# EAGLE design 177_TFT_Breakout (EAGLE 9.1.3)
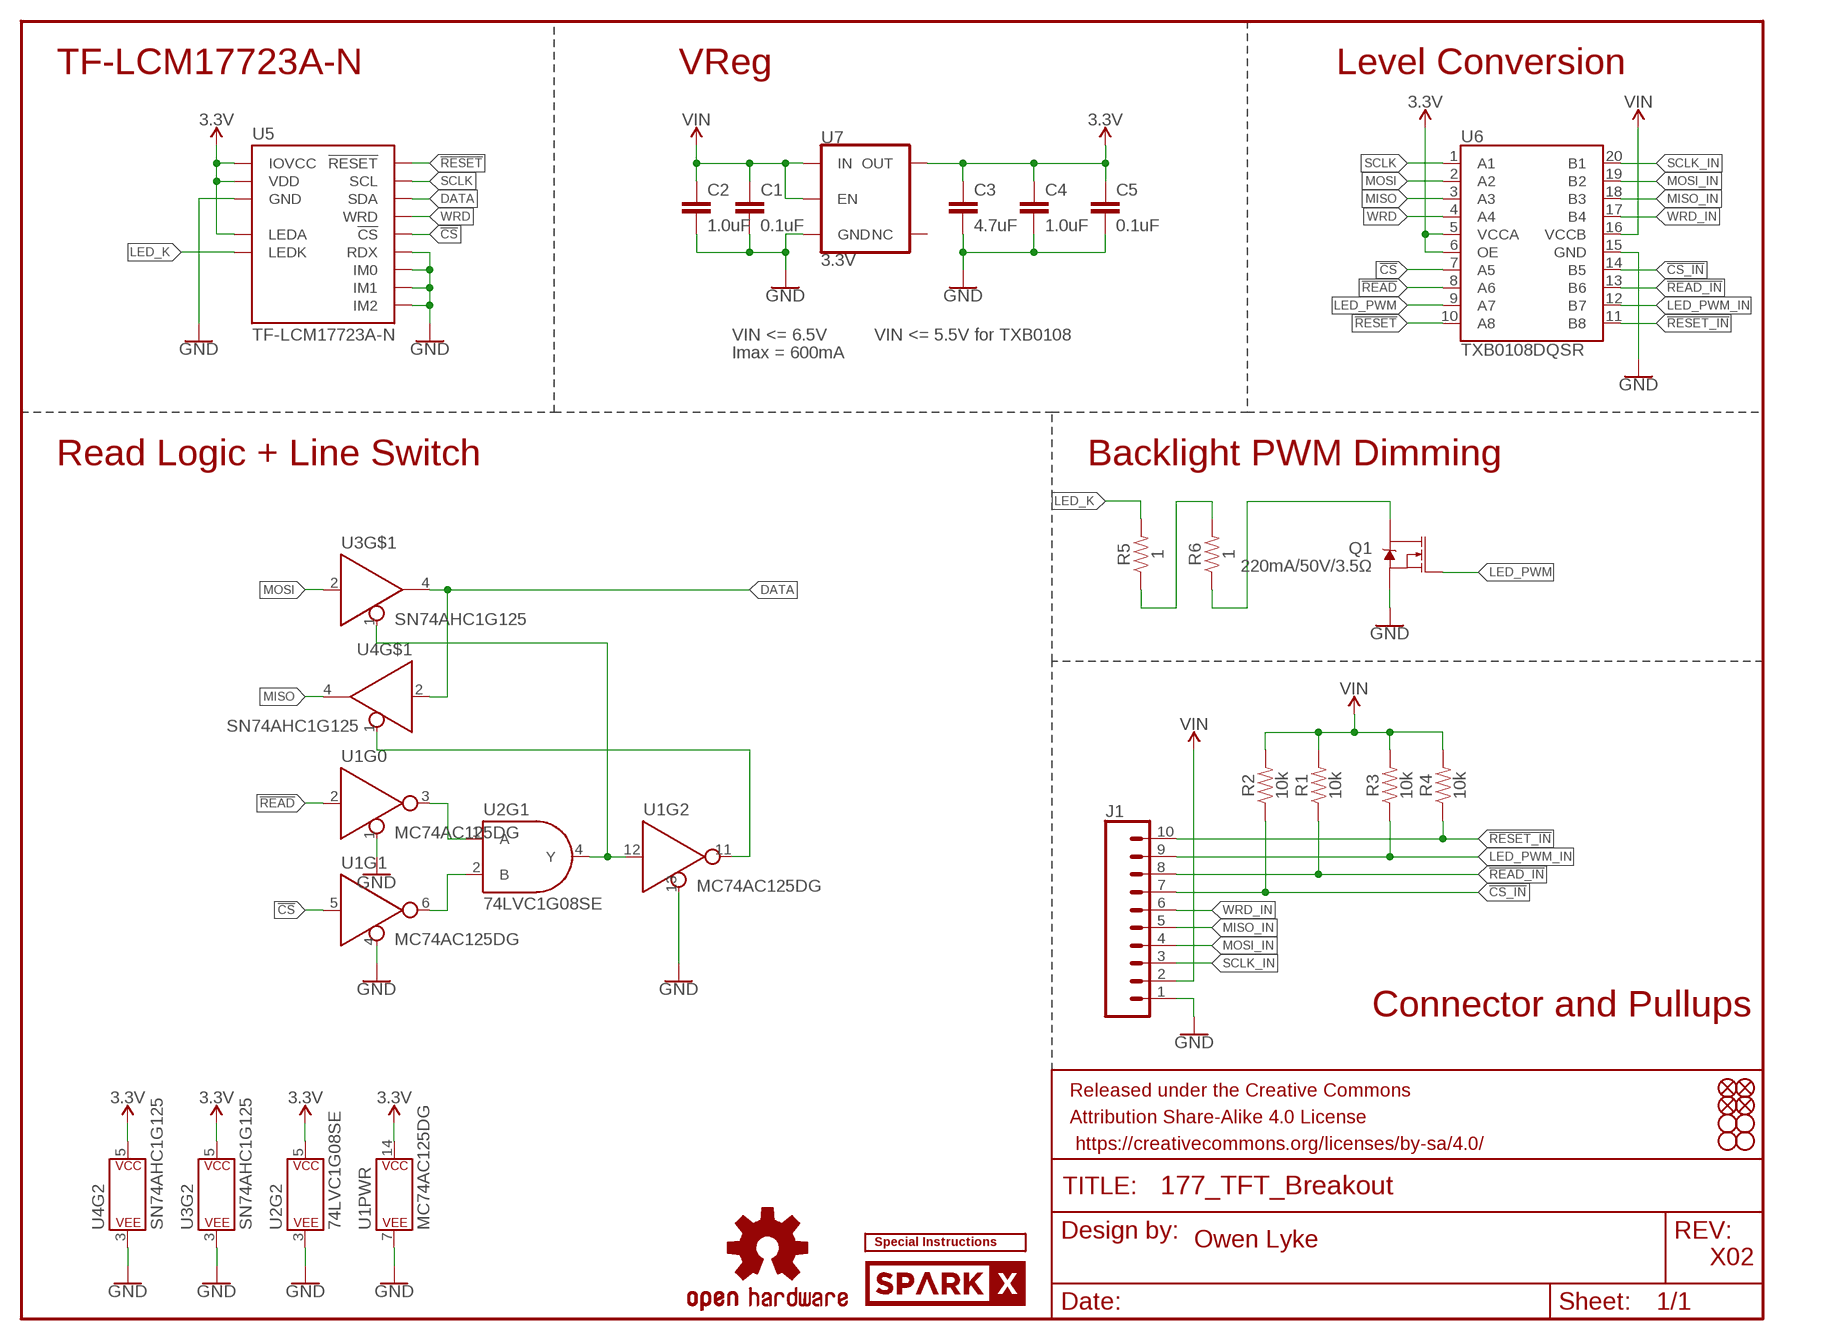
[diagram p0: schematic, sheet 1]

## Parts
C1  0.1uF  0.1UF-0603-100V-10%  [0603]
C2  1.0uF  1.0UF-0603-16V-10%  [0603]
C3  4.7uF  4.7UF-0603-6.3V-(10%)  [0603]
C4  1.0uF  1.0UF-0603-16V-10%  [0603]
C5  0.1uF  0.1UF-0603-100V-10%  [0603]
FD1  FIDUCIAL1X2  [FIDUCIAL-1X2]
FD2  FIDUCIAL1X2  [FIDUCIAL-1X2]
FD3  FIDUCIAL1X2  [FIDUCIAL-1X2]
FD4  FIDUCIAL1X2  [FIDUCIAL-1X2]
FRAME1  FRAME-LETTER  [CREATIVE_COMMONS]
H1  STAND-OFF  [STAND-OFF]
H2  STAND-OFF  [STAND-OFF]
H3  STAND-OFF  [STAND-OFF]
H4  STAND-OFF  [STAND-OFF]
J1  CONN_10NO_SILK_PTH_FEMALE  [1X10_NO_SILK]
LOGO1  OSHW-LOGOMINI  [OSHW-LOGO-MINI]
Q1  220mA/50V/3.5Ω  MOSFET-NCH-BSS138  [SOT23-3]
R1  10k  10KOHM-0603-1/10W-1%  [0603]
R2  10k  10KOHM-0603-1/10W-1%  [0603]
R3  10k  10KOHM-0603-1/10W-1%  [0603]
R4  10k  10KOHM-0603-1/10W-1%  [0603]
R5  1  1OHM-0603-1/10W-1%  [0603]
R6  1  1OHM-0603-1/10W-1%  [0603]
U1  MC74AC125DG  74AC125DG  [SO14]
U2  74LVC1G08SE  74LVC08SE  [SOT23-5]
U3  SN74AHC1G125  74AHC1G125D  [SOT23-5]
U4  SN74AHC1G125  74AHC1G125D  [SOT23-5]
U5  TF-LCM17723A-N  TF-LCM17723A-N-BOTTOM_CONTACTS  [FPC05040-17204]
U6  TXB0108DQSR  TXB0108  [UFDFN-20]
U7  3.3V  V_REG_AP2112K-3.3V  [SOT23-5]
U$26  SPECIAL_INSTRUCTIONS-ORDERING  [ORDERING_INSTRUCTIONS]
U$34  SPARKX-LOGO2  [SPARKX-TINY]

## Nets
3.3V: C3.1 C4.1 C5.1 U1.14(PWR:P$V+) U2.5(P$V+) U3.5(P$V+) U4.5(P$V+) U5.P$8(LEDA) U5.P$9(VDD) U5.P$10(IOVCC) U6.5(VCCA) U6.6(OE) U7.5(OUT)
!CS: U1.5(A) U5.P$35(!CS) U6.7(A5)
!CS_IN: J1.7 R2.1 U6.14(B5)
!READ: U1.2(A) U6.8(A6)
!READ_IN: J1.8 R1.1 U6.13(B6)
!RESET: U5.P$37(!RESET) U6.10(A8)
!RESET_IN: J1.10 R4.1 U6.11(B8)
DATA: U3.4(Y) U4.2(A) U5.P$29(SDA) U5.P$31(SDA)
GND: C1.2 C2.2 C3.2 C4.2 C5.2 J1.1 Q1.2(S) U1.1(!EN) U1.4(!EN) U1.7(PWR:P$V-) U1.13(!EN) U2.3(P$V-) U3.3(P$V-) U4.3(P$V-) U5.P$1(GND) U5.P$2(GND) U5.P$3(GND) U5.P$4(GND) U5.P$11(GND) U5.P$12(GND) U5.P$13(GND) U5.P$32(RDX) U5.P$38(IM0) U5.P$39(IM1) U5.P$40(IM2) U6.15(GND) U7.2(GND)
LED_K: R5.2 U5.P$6(LEDK) U5.P$7(LEDK)
LED_PWM: Q1.1(G) U6.9(A7)
LED_PWM_IN: J1.9 R3.1 U6.12(B7)
MISO: U4.4(Y) U6.3(A3)
MISO_IN: J1.5 U6.18(B3)
MOSI: U3.2(A) U6.2(A2)
MOSI_IN: J1.4 U6.19(B2)
N$1: U1.6(Y) U2.2(B)
N$2: U1.3(Y) U2.1(A)
N$3: U1.12(A) U2.4(Y) U3.1(!EN)
N$4: R5.1 R6.2
N$5: Q1.3(D) R6.1
N$8: U1.11(Y) U4.1(!EN)
SCLK: U5.P$34(SCL) U6.1(A1)
SCLK_IN: J1.3 U6.20(B1)
VIN: C1.1 C2.1 J1.2 R1.2 R2.2 R3.2 R4.2 U6.16(VCCB) U7.1(IN) U7.3(EN)
WRD: U5.P$33(WRD) U6.4(A4)
WRD_IN: J1.6 U6.17(B4)
Unconnected: U1.8(Y) U1.9(A) U1.10(!EN) U7.4(NC)

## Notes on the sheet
- TF-LCM17723A-N | VReg | Level Conversion
- VIN <= 6.5V | VIN <= 5.5V for TXB0108
- Imax = 600mA
- Read Logic + Line Switch | Backlight PWM Dimming
- Connector and Pullups
- Owen Lyke
- X02

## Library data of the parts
C1 C5 = SparkFun-Capacitors:0.1UF: 0.1µF ceramic capacitors; PROD_ID: CAP-08390
C2 C4 = SparkFun-Capacitors:1.0UF: 1µF ceramic capacitors; PROD_ID: CAP-00868
C3 = SparkFun-Capacitors:4.7UF: 4.7µF ceramic capacitors; PROD_ID: CAP-08280
FD1-FD4 = SparkFun-Aesthetics:FIDUCIAL: Fiducial Alignment Points
FRAME1 = SparkFun-Aesthetics:FRAME-LETTER: Schematic Frame - Letter
H1-H4 = SparkFun-Hardware:STAND-OFF: Stand Off
J1 = SparkFun-Connectors:CONN_10: Multi connection point. Often used as Generic Header-pin footprint for 0.1 inch spaced/style header connections On any of the 0.1 inch spaced packages, you can populate with these: Break Away Headers - Straight (PRT-00116) Break Away Male Headers - Right Angle (PRT-00553) Female Headers (PRT-00115)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; PROD_ID: CONN-11563
LOGO1 = SparkFun-Aesthetics:OSHW-LOGO: Open-Source Hardware (OSHW) Logo
Q1 = SparkFun-DiscreteSemi:MOSFET-NCH: N-channel MOSFETs Voltage controlled devices that allow control of high current outputs. SparkFun Products: SparkFun OpenScale SparkFun Digital Sandbox SparkFun Monster Moto Shield SparkFun MOSFET Power Controller; PROD_ID: TRANS-00830
R1-R4 = SparkFun-Resistors:10KOHM: 10kΩ resistor; PROD_ID: RES-00824
R5 R6 = SparkFun-Resistors:1OHM: 1Ω resistor; PROD_ID: RES-08269
U1 = SparkFun-IC-Logic:74*125: Quad inverter with enable BUFF TRI-ST QD N-INV 14SOIC SparkFun Products Pocket AVR Programmer (PGM-09825) SparkFun Line Follower Array (SEN-13582); PROD_ID: IC-08880
U2 = SparkFun-IC-Logic:74*08: Single AND gate IC GATE AND SNGL 2INPUT SOT353 SparkFun Products SparkFun LogicBlocks Kit (KIT-11006) SparkFun RedBot Mainboard (ROB-12097); PROD_ID: IC-10841
U3 U4 = SparkFun-IC-Logic:74*1G125: Single buffer Buffers & Line Drivers Tri-State Single Bus SOT-23-5 Datasheet SparkFun Products SparkFun SAMD21 Mini Breakout (DEV-13664) SparkFun SAMD21 Dev Breakout (DEV-13672) SparkFun MIDI Shield (DEV-12898) SparkFun WiFi Shield - CC3000 (DEV-12071); PROD_ID: IC-11920
U5 = all_displays:TF-LCM17723A-N
U6 = SparkFun-IC-Comms:TXB0108: 8-Bit Bi-Directional Level Shifter 1.2V-3.6V (VCCA) to 1.65V-5.5V (VCCB) bi-directional level shifter with auto direction sensing. Max data rate - VCCA 1.2V: 20Mbps (50ns), VCCA 3.3V: 100Mbps (10ns) Digikey: 296-27217-1-ND (20-UFDFN) SparkFun Products SparkFun GPS Logger Shield (GPS-13750) SparkFun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; PROD_ID: IC-12292
U7 = SparkFun-IC-Power:V_REG_AP2112: AP2112 - 600mA CMOS LDO Regulator w/ Enable The AP2112 is CMOS process low dropout linear regulator with enable function, the regulator delivers a guaranteed 600mA (min.) continuous load current. Features Output Voltage Accuracy: ±1.5% Output Current: 600mA (Min.) Foldback Short Current Protection: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; PROD_ID: VREG-12457
U$26 = SparkFun-Aesthetics:SPECIAL_INSTRUCTIONS: Special Ordering/Production Instructions Alert
U$34 = SparkX:SPARKX-LOGO

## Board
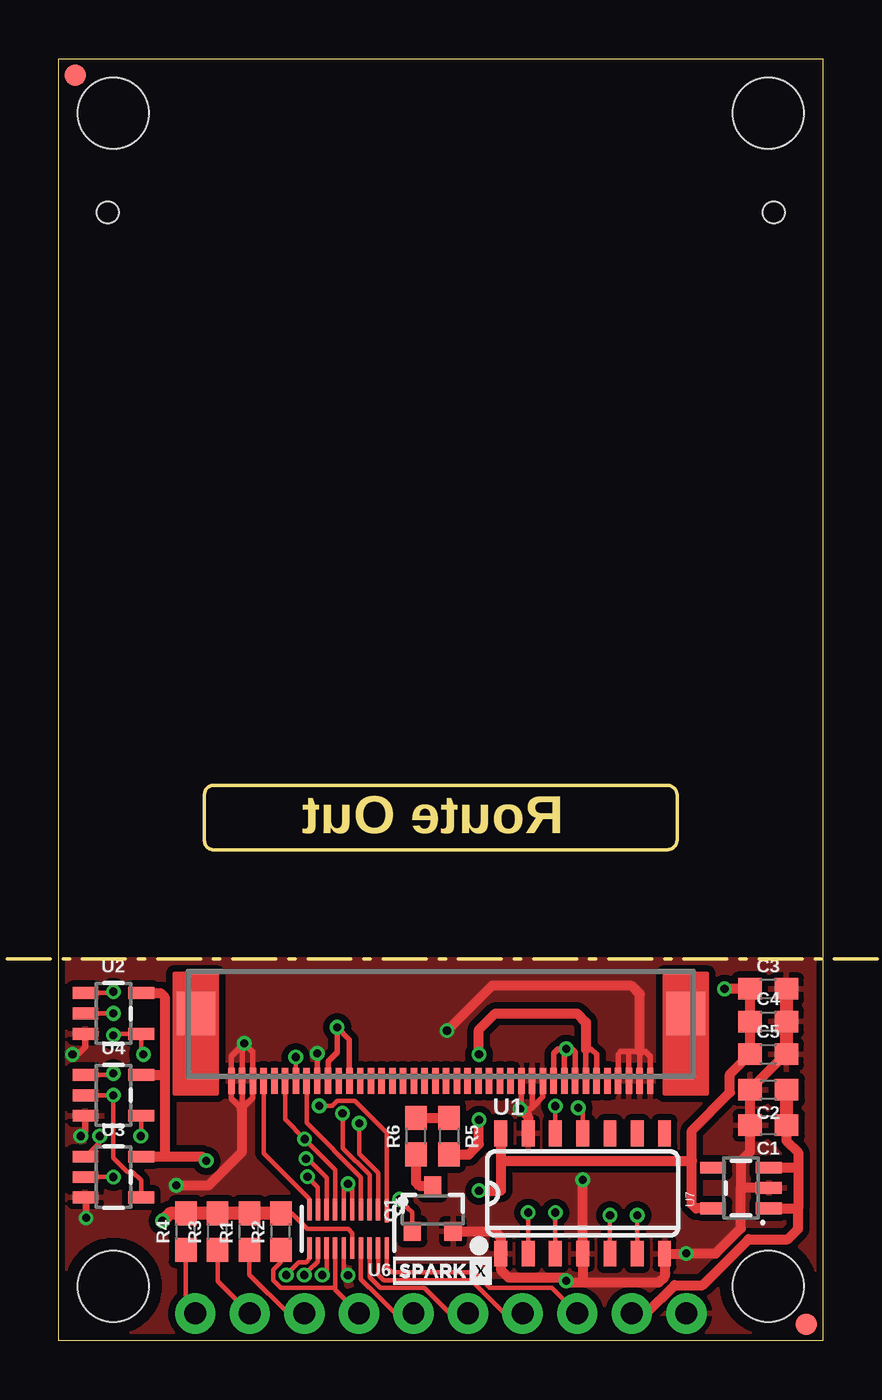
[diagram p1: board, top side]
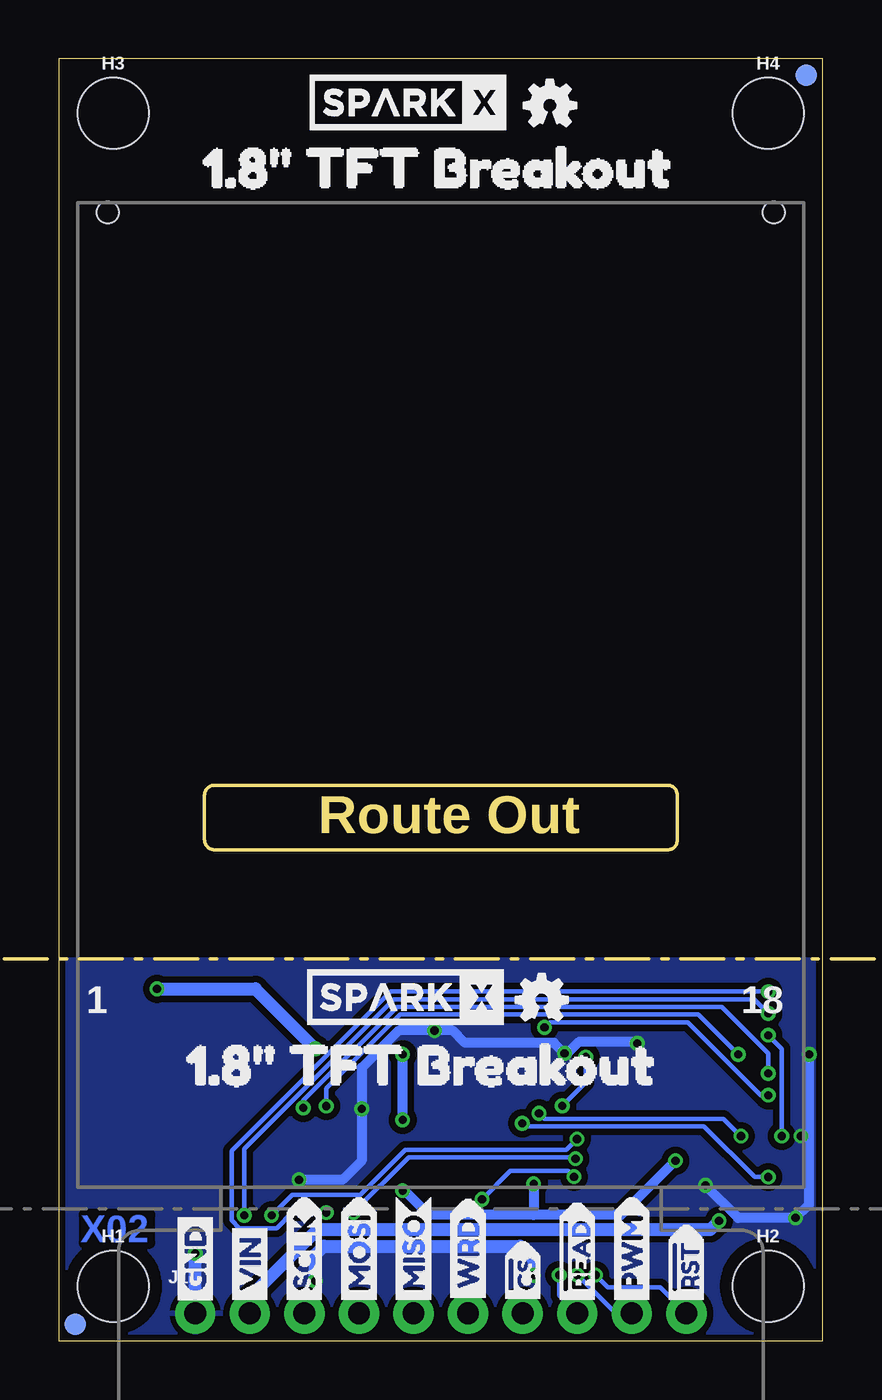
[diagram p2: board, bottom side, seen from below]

Size 35.56 x 59.69 mm. Coordinates in mm from the lower left corner, seen from the top.
Outline: 35.56,0 0,0 0,59.69 35.56,59.69 35.56,0
Copper layers (1*16): Top 0.035mm / dielectric 1.5mm / Bottom 0.035mm
Design rules "SparkFun-2-layer-PCBWay-LIMIT": minimum track width 6mil, minimum drill 0.3mm, track to track 6mil, track to pad 6mil, pad to pad 6mil, via to via 6mil, smd to smd 6mil, copper to edge 6mil, drill to drill 6mil, minimum pad ring 6mil, minimum via ring 6mil, stop-mask expansion 4mil, vias tented up to drill 25mil, thermal gap 10mil
Milling: 31 lines

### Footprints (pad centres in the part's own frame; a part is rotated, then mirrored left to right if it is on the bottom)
0603 = smd 1.1 x 1: 1 -0.85,0; 2 0.85,0
FIDUCIAL-1X2 = smd 1 x 1: 1 0,0
STAND-OFF = hole 3.302: 0,0
1X10_NO_SILK = drill 1.016 pad 1.88: 1 0,0; 2 2.54,0; 3 5.08,0; 4 7.62,0; 5 10.16,0; 6 12.7,0; 7 15.24,0; 8 17.78,0; 9 20.32,0; 10 22.86,0
SOT23-3 = smd 0.8 x 0.9: 1 -0.95,-1; 2 0.95,-1; 3 0,1.1
SO14 = smd 0.6 x 1.2: 1 -3.175,-2.8; 2 -1.905,-2.8; 3 -0.635,-2.8; 4 0.635,-2.8; 5 1.905,-2.8; 6 3.175,-2.8; 7 4.445,-2.8; 8 4.445,2.8; 9 3.175,2.8; 10 1.905,2.8; 11 0.635,2.8; 12 -0.635,2.8; 13 -1.905,2.8; 14 -3.175,2.8
SOT23-5 = smd 0.55 x 1.2: 1 -0.95,-1.3; 2 0,-1.3; 3 0.95,-1.3; 4 0.95,1.3; 5 -0.95,1.3
FPC05040-17204 = smd 0.3 x 1.2: P$1 -9.75,0.6; P$2 -9.25,0.6; P$3 -8.75,0.6; P$4 -8.25,0.6; P$5 -7.75,0.6; P$6 -7.25,0.6; P$7 -6.75,0.6; P$8 -6.25,0.6; P$9 -5.75,0.6; P$10 -5.25,0.6; P$11 -4.75,0.6; P$12 -4.25,0.6; P$13 -3.75,0.6; P$14 -3.25,0.6; P$15 -2.75,0.6; P$16 -2.25,0.6; P$17 -1.75,0.6; P$18 -1.25,0.6; P$19 -0.75,0.6; P$20 -0.25,0.6; P$21 0.25,0.6; P$22 0.75,0.6; P$23 1.25,0.6; P$24 1.75,0.6; P$25 2.25,0.6; P$26 2.75,0.6; P$27 3.25,0.6; P$28 3.75,0.6; P$29 4.25,0.6; P$30 4.75,0.6; P$31 5.25,0.6; P$32 5.75,0.6; P$33 6.25,0.6; P$34 6.75,0.6; P$35 7.25,0.6; P$36 7.75,0.6; P$37 8.25,0.6; P$38 8.75,0.6; P$39 9.25,0.6; P$40 9.75,0.6 | smd 1.8 x 2: P$41 -11.4,-2.55; P$42 11.4,-2.55
UFDFN-20 = smd 0.2 x 1.1: 1 -1.8,-0.85 | smd 0.2 x 1: 2 -1.4,-0.9; 3 -1,-0.9; 4 -0.6,-0.9; 5 -0.2,-0.9; 6 0.2,-0.9; 7 0.6,-0.9; 8 1,-0.9; 9 1.4,-0.9; 10 1.8,-0.9; 11 1.8,0.9; 12 1.4,0.9; 13 1,0.9; 14 0.6,0.9; 15 0.2,0.9; 16 -0.2,0.9; 17 -0.6,0.9; 18 -1,0.9; 19 -1.4,0.9; 20 -1.8,0.9
TF-LCM17723A-N_FLAT = hole 1: -15.5,75.4; 15.5,75.4

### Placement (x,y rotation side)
C1  33.02,10.03 180 top
C2  33.02,11.68 180 top
C3  33.02,16.38 0 top
C4  33.02,14.86 0 top
C5  33.02,13.34 0 top
FD1  34.8,0.76 0 bottom
FD2  0.76,58.93 0 bottom
FD3  34.8,0.76 0 top
FD4  0.76,58.93 0 top
FRAME1  not placed on the board
H1  33.02,2.54 0 bottom
H2  2.54,2.54 0 bottom
H3  33.02,57.15 0 bottom
H4  2.54,57.15 0 bottom
J1  29.21,1.27 0 bottom
LOGO1  12.7,57.53 0 bottom
LOGO2  OSHW-LOGOMINI  [OSHW-LOGO-MINI]  13.08,15.88 0 bottom
Q1  17.4,6.1 0 top
R1  8.86,5.08 90 top
R2  10.34,5.08 90 top
R3  7.39,5.08 90 top
R4  5.92,5.08 90 top
R5  18.16,9.53 270 top
R6  16.64,9.53 90 top
U1  23.75,6.86 0 top
U2  2.54,15.24 270 top
U3  2.54,7.62 270 top
U4  2.54,11.43 270 top
U5  17.78,12.7 180 top
U6  13.46,5.21 180 top
U7  31.75,7.11 90 top
U$1  [TF-LCM17723A-N_FLAT]  17.78,-22.86 0 bottom
U$3  [VIN2]  26.67,1.4 90 bottom
U$4  [GND1]  29.21,1.4 90 bottom
U$5  [MOSI8]  21.59,1.4 90 bottom
U$6  [MISO9]  19.05,1.4 90 bottom
U$7  [PWM8]  8.89,1.4 90 bottom
U$8  [#READ7]  11.43,1.27 90 bottom
U$9  [#CS6]  13.97,1.27 90 bottom
U$10  [WRD9]  16.51,1.52 90 bottom
U$11  [SCLK7]  24.13,1.4 90 bottom
U$12  [#RST2]  6.35,1.27 90 bottom
U$13  [SPARKX-MEDIUM]  19.3,57.66 0 bottom
U$14  [1#8#_TFT_BREAKOUT10]  30.48,54.61 0 bottom
U$15  [1#8#_TFT_BREAKOUT10]  31.24,12.83 0 bottom
U$26  not placed on the board
U$34  17.86,3.25 0 top
U$51  [SPARKX-MEDIUM]  19.43,16 0 bottom

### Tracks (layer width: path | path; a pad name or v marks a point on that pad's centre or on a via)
3.3V  (via drill 0.38)
  Top 0.203: U6.5 13.66,7.1 v13.46,7.3 13.26,7.11 U6.6
  Top 0.254: U5.P$10 23.03,13.38 23.24,13.59 v23.62,13.59 | U5.P$9 23.53,13.5 v23.62,13.59 | v23.62,13.59 23.88,13.59 24.03,13.44 U5.P$8
  Top 0.457: v30.99,16.38 C3.1 C4.1 C5.1 31.24,12.4 31.24,11.56 29.46,9.78 29.46,8.38 | v6.86,8.38 6.67,8.57 4.95,8.57 | 4.95,8.57 U3.5 | U2.5 4.74,16.19 4.92,16 4.92,12.32 | 4.92,12.32 4.92,8.6 4.95,8.57 | U4.5 4.86,12.38 4.92,12.32 | 29.46,8.38 29.46,6.35 29.65,6.16 U7.5 | U1.14 20.57,8.38 | 20.57,8.38 20.57,6.99 v19.56,6.99 | 20.57,8.38 29.46,8.38
  Bottom 0.457: v19.56,6.99 19.52,7.03 18.34,5.86 13.46,5.86 | v6.86,8.38 9.38,5.86 13.46,5.86 | v13.46,7.3 13.46,5.86
  Bottom 0.61: v30.99,16.38 26.42,16.38 v23.62,13.59
!CS  (via drill 0.38)
  Top 0.203: v25.65,5.84 U1.5 | U5.P$35 10.53,10.3 v11.44,9.39 12.86,7.97 U6.7
  Bottom 0.203: v25.65,5.84 24.7,6.79 21.52,6.79 19.43,8.89 11.94,8.89 v11.44,9.39
!CS_IN
  Top 0.203: U6.14 12.86,2.54 | 12.86,2.54 12.86,2.38 J1.7 | 12.86,2.54 12.79,2.46 10.34,2.46 9.99,2.81 9.99,3.31 10.34,3.66 R2.1
!READ  (via drill 0.38)
  Top 0.203: v21.84,5.97 U1.2 | U6.8 12.46,7.6 11.58,8.47 v11.51,8.47
  Bottom 0.203: v21.84,5.97 19.28,8.53 11.57,8.53 v11.51,8.47
!READ_IN  (via drill 0.38)
  Top 0.203: R1.1 8.87,3.07 10.67,1.27 J1.8 | U6.13 12.46,3.26 v12.27,3.06
  Bottom 0.203: v12.27,3.06 12.27,2.1 J1.8
!RESET
  Top 0.203: U6.10 11.66,6.6 9.53,8.74 U5.P$37
!RESET_IN  (via drill 0.38)
  Top 0.203: J1.10 5.92,1.7 R4.1 | U6.11 11.66,3.81 11.52,3.66 11.18,3.66 v10.58,3.06
  Bottom 0.203: J1.10 7.56,2.48 10,2.48 v10.58,3.06
DATA  (via drill 0.38)
  Top 0.203: U4.2 v2.54,11.43 2.54,8.51 3.17,7.87 3.43,7.87 3.84,7.46 U3.4
  Top 0.254: U5.P$29 13.53,14.02 v12.95,14.59 12.95,13.43 12.53,13 U5.P$31
  Bottom 0.203: v2.54,11.43 2.88,11.43 6.28,14.83 12.71,14.83 v12.95,14.59
GND  (via drill 0.38)
  Top 0.203: U6.15 13.26,3.25 v13.46,3.05 | v12.03,13.37 v12.02,13.38
  Top 0.254: 26.54,13.46 26.16,13.46 26.03,13.33 U5.P$4 | 26.54,13.46 27.05,13.46 | 27.05,13.46 27.3,13.46 27.53,13.24 U5.P$1 | 27.05,13.46 27.03,13.44 U5.P$2 | U5.P$13 21.53,10.86 v21.46,10.79 21.97,10.79 22.03,10.85 | U5.P$11 22.53,11.35 22.03,10.85 | U5.P$12 22.03,10.85 | U5.P$32 v12.03,13.37 | v8.64,13.84 8.03,13.24 U5.P$40 8.03,11.27 8.51,10.79 8.53,10.82 | v8.64,13.84 9.03,13.45 U5.P$38 9.03,11.32 8.53,10.82 | v8.64,13.84 8.53,13.74 U5.P$39 8.53,10.82 | U5.P$3 26.53,13.45 26.54,13.46
  Top 0.305: U2.3 1.24,13.69 0.89,13.34 v0.64,13.34 | U4.3 1.24,9.75 v1.02,9.53 | U3.3 1.27,6.64 v1.27,5.71
  Top 0.457: C5.2 33.82,13.34 C2.2 C1.2 32.17,8.8 31.75,8.38 31.75,7.11 | U1.13 21.84,10.41 v21.46,10.79 | U7.2 31.75,7.11 | v5.46,7.24 6.99,7.24 8.51,8.76 8.51,10.79 | 24.38,2.7 27.91,2.7 28.19,2.98 U1.7 v29.2,4.06 v29.21,4.06 30.58,4.06 31.75,5.23 31.75,7.11 | 24.38,2.7 23.72,2.7 v23.62,2.79 23.47,2.95 20.93,2.95 20.57,3.3 U1.1 20.57,4.83 20.3,5.1 Q1.2 | 24.38,2.7 U1.4 v24.38,7.49 | 27.05,13.46 27.05,16.13 26.67,16.51 20.14,16.51 v18.07,14.44
  Top 0.61: C3.2 C4.2 C5.2
  Bottom 0.457: 0.64,9.53 0.64,6.35 v1.27,5.71 3.94,5.71 v5.46,7.24 | 0.64,9.53 v0.64,13.34 | v1.02,9.53 0.64,9.53 | v8.64,13.84 8.72,13.93 11.33,13.93 11.89,13.38 v12.02,13.38 12.52,13.87 16.66,13.87 17.23,14.44 v18.07,14.44 19.74,14.44 21.46,12.71 v21.46,10.79 21.46,8.38 22.35,7.49 v24.38,7.49
  Bottom 0.61: J1.1 v29.21,4.06 | v23.62,2.79 23.62,4 23.22,4.41 14.1,4.41 13.46,3.77 v13.46,3.05
  pour Top (isolate 0.305): 0,0 0,17.78 35.56,17.78 35.56,0
  pour Bottom (isolate 0.305): 0,0 0,17.78 35.56,17.78 35.56,0
LED_K  (via drill 0.38)
  Top 0.254: U5.P$7 24.53,13.56 24.54,13.56 24.79,13.56 25.03,13.32 U5.P$6
  Top 0.457: 24.54,13.56 24.54,14.83 24.13,15.24 20.32,15.24 19.56,14.48 v19.56,13.34 | R5.2 19.09,8.68 19.56,9.14 v19.56,10.29
  Bottom 0.457: v19.56,10.29 v19.56,13.34
LED_PWM  (via drill 0.38)
  Top 0.203: Q1.1 16.45,5.97 16.23,6.19 16.23,6.21 v15.86,6.58 | U6.9 12.06,7.15 v11.58,7.64
  Bottom 0.203: v15.86,6.58 14.54,7.9 11.84,7.9 v11.58,7.64
LED_PWM_IN  (via drill 0.38)
  Top 0.203: J1.9 7.39,2.77 R3.1 | v11.43,3.06 11.67,3.3 11.67,3.31 12.02,3.66 12.06,3.7 U6.12
  Bottom 0.203: v11.43,3.06 9.64,1.27 J1.9
MISO  (via drill 0.38)
  Top 0.203: v3.81,9.53 3.84,9.55 U4.4 | U6.3 14.46,7.71 13.21,8.97 v13.21,10.58
  Bottom 0.203: v3.81,9.53 4.62,10.34 12.97,10.34 v13.21,10.58
MISO_IN
  Top 0.203: U6.18 14.46,2.96 14.61,2.82 14.97,2.46 17,2.46 18.2,1.27 J1.5
MOSI  (via drill 0.38)
  Top 0.203: v2.54,7.62 U3.2 | U6.2 14.86,7.82 13.98,8.69 v13.98,10.12
  Bottom 0.203: v2.54,7.62 3.17,7.62 5.54,9.98 13.85,9.98 v13.98,10.12
MOSI_IN
  Top 0.203: U6.19 14.86,3.07 15.12,2.82 19.19,2.82 20.74,1.27 J1.4
N$1  (via drill 0.38)
  Top 0.203: U2.2 v2.54,15.24 | v26.92,5.84 U1.6
  Bottom 0.203: v2.54,15.24 3.2,15.9 19.96,15.9 26.92,8.94 v26.92,5.84
N$2  (via drill 0.38)
  Top 0.203: U2.1 2.47,16.19 v2.54,16.26 | v23.11,5.97 U1.3
  Bottom 0.203: v23.11,5.97 24.68,5.97 25.41,5.25 27.17,5.25 27.52,5.59 27.52,8.85 20.11,16.26 v2.54,16.26
N$3  (via drill 0.38)
  Top 0.203: v2.54,14.22 2.61,14.29 U2.4 3.84,13.43 v3.94,13.34 | v23.11,10.92 U1.12 | U3.1 1.91,9.23 v1.91,9.53
  Bottom 0.203: v3.94,13.34 5.79,15.19 19.67,15.19 23.11,11.74 v23.11,10.92 | v1.91,9.53 1.91,13.59 v2.54,14.22
N$4
  Top 0.457: R6.2 R5.1
N$5
  Top 0.457: Q1.3 16.81,7.2 16.64,7.37 R6.1
N$8  (via drill 0.38)
  Top 0.203: U4.1 2.47,12.38 v2.54,12.45 | U1.11 24.38,10.64 v24.18,10.84
  Bottom 0.203: v2.54,12.45 2.54,13.38 4.71,15.54 19.82,15.54 24.18,11.18 v24.18,10.84
SCLK  (via drill 0.38)
  Top 0.203: U5.P$34 v11.03,13.21 | U6.1 15.26,9.69 13.77,11.18 12.96,11.18 12.72,10.94 v12.13,10.94
  Bottom 0.203: v12.13,10.94 11.03,12.03 v11.03,13.21
SCLK_IN
  Top 0.203: U6.20 15.26,3.43 15.52,3.17 19.34,3.17 20.05,2.46 22.94,2.46 J1.3
VIN  (via drill 0.38)
  Top 0.203: U6.16 13.66,5.01 13.46,5.21 11.56,5.21 10.83,5.93 R2.2
  Top 0.457: J1.2 27.34,1.27 28.66,2.59 29.97,2.59 32.1,4.72 33.93,4.72 34.42,5.21 34.42,6.16 | U7.3 34.42,8.06 | 34.42,8.06 34.42,6.16 | C1.1 33.87,9.31 34.42,8.76 34.42,8.06 | U7.1 34.42,6.16
  Top 0.61: R2.2 R1.2 R3.2 R4.2 5.18,5.93 v4.83,5.58 | C2.1 C1.1
  Bottom 0.61: J1.2 26.67,2.03 23.53,5.17 5.25,5.17 v4.83,5.58
WRD
  Top 0.203: U6.4 14.06,7.61 11.53,10.14 U5.P$33
WRD_IN
  Top 0.203: J1.6 15.66,1.27 14.46,2.46 14.06,2.86 U6.17

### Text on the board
Bottom: X02
Dimension: Route Out
bPlace: 18 | 1
Reference: Score here for compact breakout
bDocu: When panelizing this file ensure that the v-score lines for the / breakaway portion are continued across the whole panel, and labeled | Owen Lyke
